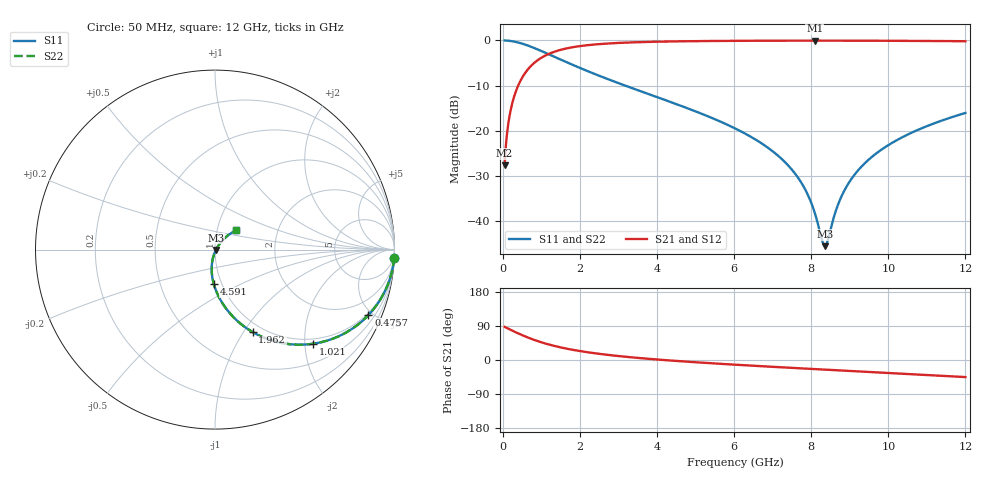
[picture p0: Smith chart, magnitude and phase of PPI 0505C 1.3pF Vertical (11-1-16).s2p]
# GHz S MA R 50
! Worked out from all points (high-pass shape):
!   1601 points, 50 MHz to 12 GHz, reference 50 ohm
!   highest |S21| = -0.05 dB at 8.094 GHz (marker M1); lowest = -27.6 dB at 50 MHz (marker M2)
!   |S21| within 3 dB of the highest: 1.177 GHz to end of sweep
!   lowest |S11| = -45.5 dB at 8.355 GHz (marker M3), VSWR 1.01, Z = 50.5 - j0.243 ohm
!   |S11| at or under -10 dB: 3.181 GHz to end of sweep
!   |S22| runs from -45.5 to 0.0 dB; largest |S21 - S12| = 0
!   S11 on the Smith chart (normalised r, x): 50 MHz: 1, -45; 475.7 MHz: 0.89, -4.74; 1.021 GHz: 0.89, -2.19; 1.962 GHz: 0.89, -1.10; 4.591 GHz: 0.92, -0.36; 12 GHz: 1.23, +0.27
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0.05  0.9991 -2.5  0.0415 87.5  0.0415 87.5  0.9991 -2.5
0.1470937  0.9926 -7.4  0.1213 82.6  0.1213 82.6  0.9926 -7.4
0.2217813  0.9834 -11.1  0.1813 78.9  0.1813 78.9  0.9834 -11.1
0.4757188  0.9294 -23.1  0.3682 66.9  0.3682 66.9  0.9294 -23.1
1.020938  0.7582 -43.8  0.6505 46.1  0.6505 46.1  0.7582 -43.8
1.962  0.5052 -65.5  0.8605 24.3  0.8605 24.3  0.5052 -65.5
2.044156  0.4884 -66.8  0.87 22.9  0.87 22.9  0.4884 -66.8
2.888125  0.3519 -77.8  0.9329 11.7  0.9329 11.7  0.3519 -77.8
4.038312  0.2334 -88.1  0.9686 1.0  0.9686 1.0  0.2334 -88.1
4.591  0.1916 -92.0  0.9774 -3.1  0.9774 -3.1  0.1916 -92.0
6.025  0.1067 -100.0  0.9895 -12.4  0.9895 -12.4  0.1067 -100.0
7.309625  0.04573 -103.6  0.9936 -19.7  0.9936 -19.7  0.04573 -103.6
7.720406  0.02784 -101.5  0.9941 -22.0  0.9941 -22.0  0.02784 -101.5
8.019156  0.01538 -93.9  0.9942 -23.6  0.9942 -23.6  0.01538 -93.9
8.093844  0.01242 -89.2  0.9942 -24.0  0.9942 -24.0  0.01242 -89.2
8.35525  0.005328 -26.9  0.9941 -25.4  0.9941 -25.4  0.005328 -26.9
8.429937  0.006157 3.7  0.9941 -25.8  0.9941 -25.8  0.006157 3.7
8.71375  0.016 42.6  0.9939 -27.4  0.9939 -27.4  0.016 42.6
8.982625  0.02694 49.2  0.9935 -28.8  0.9935 -28.8  0.02694 49.2
9.415812  0.04497 51.5  0.9926 -31.1  0.9926 -31.1  0.04497 51.5
10.01331  0.07018 50.7  0.9908 -34.3  0.9908 -34.3  0.07018 50.7
12  0.158 42.4  0.9796 -45.0  0.9796 -45.0  0.158 42.4
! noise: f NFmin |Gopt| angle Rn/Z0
0.05  0.001017  0.9623  1.63  0.006095
1.372  0.005841  0.7682  6.002  0.005116
2.701  0.00922  0.7174  9.677  0.006406
4.031  0.01221  0.6874  13.44  0.007487
5.36  0.01502  0.6674  17.19  0.008485
6.682  0.01775  0.6538  20.87  0.009457
8.012  0.02049  0.6449  24.52  0.01046
9.341  0.02329  0.6397  28.09  0.01152
10.67  0.02618  0.6378  31.59  0.01267
12  0.02922  0.6388  35.02  0.01395
